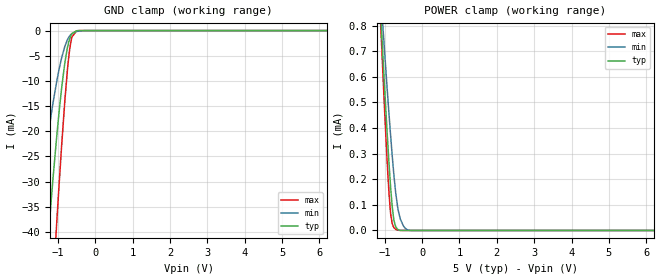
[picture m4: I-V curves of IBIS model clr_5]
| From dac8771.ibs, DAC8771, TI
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|   clr_5 Model
[Model]   clr_5
Model_type   Input
Vinl = 0.8
Vinh = 2
|   typ   min   max
|   (nom PVT)   (fast PVT)   (slow PVT)
C_comp   8.232e-13   7.943e-13   8.537e-13
| Where nom  PVT is Nominal Process, 5V, 27C
|   Fast PVT is Strong Process,  5.5V, -40C
|   Slow PVT is Weak Process,   4.5V, 150C
[Voltage Range]   5   4.5   5.5
|Junction Temperature
[Temperature Range]   27   150   -40
[Power Clamp Reference]   5   4.5   5.5
[GND Clamp Reference]   0   0   0
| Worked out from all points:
|   GND clamp passes 1 mA (typ) near -0.65 V on its own axis
|   POWER clamp passes 1 mA (typ) near -1.16 V on its own axis
[GND Clamp]
|   Voltage   I(typ)   I(min)   I(max)
-5V       -474.9mA   -340.4mA   -567mA
-1.769V   -94.94mA   -52.74mA   -135.2mA
-1.546V   -70.71mA   -37.79mA   -105.4mA
-1.328V   -48.29mA   -24.72mA   -76.5mA
-1.17V    -33.26mA   -16.46mA   -56.01mA
-1.115V   -28.36mA   -13.87mA   -49.03mA
-1.03V    -21.24mA   -10.21mA   -38.5mA
-815mV    -6.672mA   -3.257mA   -14.41mA
-710mV    -2.383mA   -1.387mA   -5.538mA
-620mV    -629.9uA   -578.5uA   -1.271mA
-500mV    -47.18uA   -184.6uA   -68.85uA
10V       0A         0A         0A
[POWER Clamp]
|   Voltage   I(typ)   I(min)   I(max)
-5V       12.66mA    10.18mA    14.82mA
-1.099V   825.6uA    909.4uA    780.8uA
-1.007V   574.8uA    711.1uA    488.1uA
-914mV    335.5uA    517uA      220.7uA
-850mV    189.9uA    390.3uA    82.88uA
-798mV    95.78uA    294.2uA    27.83uA
-750mV    40.4uA     213.7uA    11.12uA
-644mV    3.039uA    83.89uA    1.12uA
-581mV    429nA      44.71uA    188.2nA
-500mV    33.02nA    18.58uA    12.26nA
-310mV    0A         383.3nA    0A
10V       0A         0A         0A
